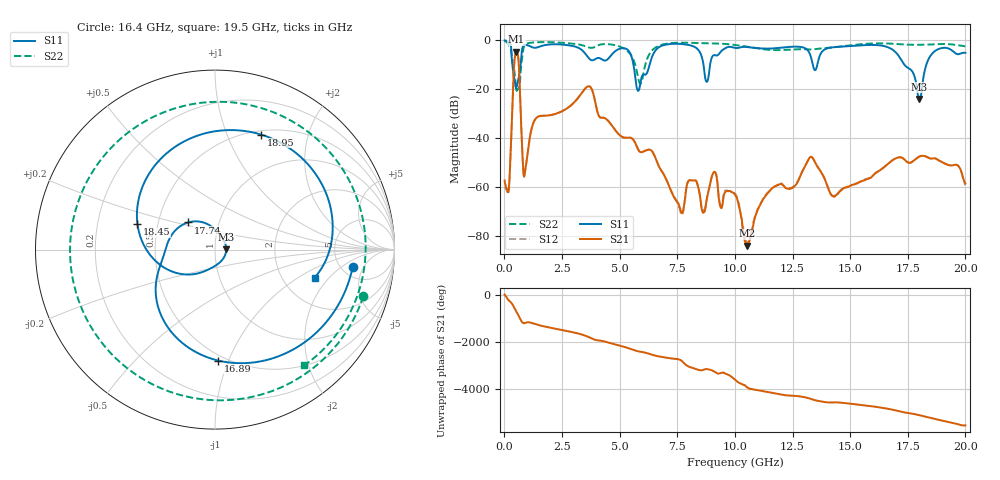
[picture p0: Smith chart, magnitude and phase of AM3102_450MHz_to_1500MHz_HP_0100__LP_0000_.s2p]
!Agilent Technologies,E8364B,MY43040894,A.07.50.67
!Agilent E8364B: A.07.50.67
!Date: Thursday, January 11, 2018 05:34:42
!Correction: S11(Full 2 Port(1,2))
!S21(Full 2 Port(1,2))
!S12(Full 2 Port(1,2))
!S22(Full 2 Port(1,2))
!S2P File: Measurements: S11, S21, S12, S22:
# Hz S  dB  R 50
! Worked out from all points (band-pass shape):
!   1601 points, 10 MHz to 20 GHz, reference 50 ohm
!   highest |S21| = -4.65 dB at 522.2 MHz (marker M1); lowest = -84.1 dB at 10.52 GHz (marker M2)
!   |S21| within 3 dB of the highest: 445.7 MHz to 608.2 MHz (162.4 MHz wide, 30.8 % of centre)
!   lowest |S11| = -24.1 dB at 18 GHz (marker M3), VSWR 1.13, Z = 56.7 + j0.128 ohm
!   |S11| at or under -10 dB: 345.4 MHz to 703 MHz (357.6 MHz wide, 68.2 % of centre); 5.601 GHz to 6.299 GHz (698.5 MHz wide, 11.7 % of centre); 17.35 GHz to 18.3 GHz (950.7 MHz wide, 5.33 % of centre)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
!   |S22| runs from -20.7 to -0.3 dB; largest |S21 - S12| = 0.0021
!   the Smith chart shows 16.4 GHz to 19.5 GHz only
!   S11 on the Smith chart (normalised r, x): 16.4 GHz: 6.30, -3.06; 16.89 GHz: 0.46, -0.92; 17.74 GHz: 0.71, +0.23; 18.45 GHz: 0.38, +0.14; 18.95 GHz: 0.54, +1.33; 19.5 GHz: 3.00, -1.40
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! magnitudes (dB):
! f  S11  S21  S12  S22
! 10 MHz  -0.1  -57.4  -60.0  -0.3
! 197.4 MHz  -0.7  -60.2  -61.0  -2.4
! 522.2 MHz  -18.7  -4.7  -4.7  -20.5
! 884.6 MHz  -1.9  -54.6  -54.5  -2.0
! 1.359 GHz  -3.0  -32.1  -32.1  -0.8
! 3.346 GHz  -3.9  -21.7  -21.7  -1.9
! 5.807 GHz  -20.7  -44.7  -44.8  -15.5
! 6.682 GHz  -3.0  -51.2  -51.2  -2.3
! 7.669 GHz  -1.5  -70.6  -71.3  -1.0
! 10.01 GHz  -3.1  -63.2  -62.8  -1.9
! 10.52 GHz  -2.8  -84.1  -83.1  -2.6
! 13.34 GHz  -8.4  -47.8  -47.8  -3.8
! 14.28 GHz  -2.8  -63.9  -63.8  -2.9
! 16.4 GHz  -2.2  -52.5  -52.4  -1.2
! 16.68 GHz  -3.0  -50.3  -50.3  -1.3
! 16.89 GHz  -4.2  -48.8  -48.8  -1.4
! 17.74 GHz  -13.5  -49.4  -49.4  -1.9
! 18 GHz  -24.1  -47.6  -47.6  -1.9
! 18.45 GHz  -6.9  -48.3  -48.3  -1.7
! 18.95 GHz  -3.2  -49.7  -49.7  -1.5
! 19.5 GHz  -4.8  -51.1  -51.1  -1.8
! 20 GHz  -5.1  -58.7  -59.3  -2.4
